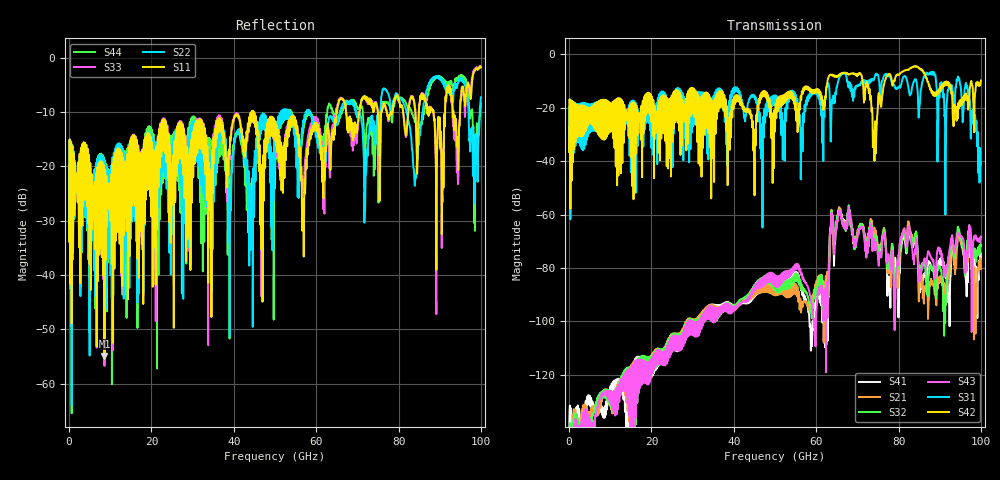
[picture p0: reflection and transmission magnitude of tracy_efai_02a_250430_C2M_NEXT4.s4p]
!! PART DESCRIPTION: TE 224G+ VSR Channel- Chip to module, IO connector to CPC(Co-packaged connector) through over the board cable
!! CHANNEL DESCRIPTION: Module trace -> Mated IO 224G+ Connector -> Internal Cable Termination -> 30AWG 300mm Cable -> Cable
!!  termination + CPC connector(No footprint or package included)
!! MODEL REVISION:  Rev 3, Created on April 29, 2025
!! MODEL STATUS: Development
!! MODEL GEOMETRY: NEXT4
!! MODEL FREQUENCY RANGE: 0 GHz to 100 GHz in 10.00 MHz frequency steps
!! PORT DEFINITIONS:
!! Port  1  ----->  Module Side  -->  Module Side  <-----  Port  2
!! Port  3  ----->  Module Side  -->  Module Side  <-----  Port  4
# HZ S MA R 45.000000
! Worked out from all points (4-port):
!   10000 points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, 10 MHz to 100 GHz, reference 45 ohm
!   strongest paths, dB at 10 MHz, 25.01 GHz, 50.01 GHz, 75.01 GHz, 100 GHz:
!     S42: -36.6, -18.4, -28.2, -17.6, -9.8
!     S31: -36.5, -17.8, -16.0, -7.7, -40.6
!     S43: -150.2, -111.0, -83.2, -75.4, -68.2
!     S32: -149.5, -109.9, -84.2, -73.0, -71.6
!     S21: -150.1, -109.9, -85.2, -72.8, -80.3
!     S41: -147.7, -110.5, -84.1, -73.3, -76.5
!   lowest |S11| = -54.9 dB at 8.6 GHz (marker M1), VSWR 1.00, Z = 44.9 + j0.15 ohm
!   |S11| at or under -10 dB: start of sweep to 44.32 GHz; 44.72 GHz to 64.9 GHz (20.18 GHz wide, 36.8 % of centre); 67.23 GHz to 70.41 GHz (3.185 GHz wide, 4.63 % of centre)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
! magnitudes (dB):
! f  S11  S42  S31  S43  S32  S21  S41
! 10 MHz  -33.8  -36.6  -36.5  -150.2  -149.5  -150.1  -147.7
! 8.6 GHz  -54.9  -28.6  -27.5  -127.3  -127.6  -127.9  -136.1
! 62.64 GHz  -13.7  -11.2  -12.0  -86.2  -89.6  -82.2  -88.9
! 65.68 GHz  -7.8  -7.5  -8.4  -59.1  -58.3  -57.7  -58.5
! 74.21 GHz  -8.4  -32.3  -8.5  -72.2  -68.9  -66.4  -69.0
! 88.17 GHz  -9.4  -13.7  -7.5  -76.5  -79.6  -84.9  -80.2
! 100 GHz  -1.8  -9.8  -40.6  -68.2  -71.6  -80.3  -76.5
